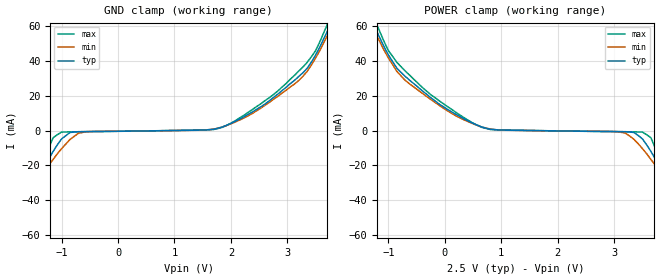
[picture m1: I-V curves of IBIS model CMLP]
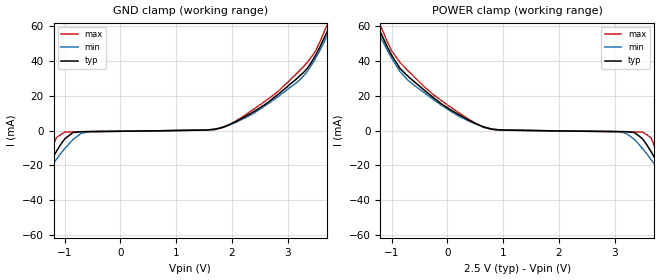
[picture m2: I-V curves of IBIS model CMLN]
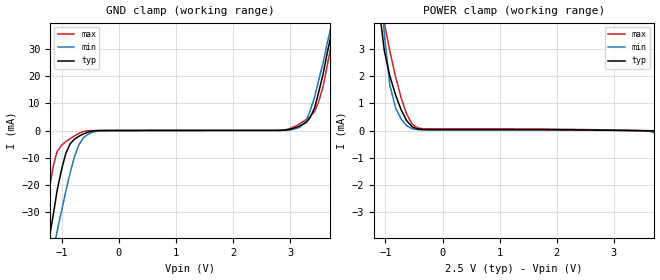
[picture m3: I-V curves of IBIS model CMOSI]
|   Texas Instruments Incorporated
|   IBIS Model of DS30EA101
[IBIS Ver]   4.2
[File name]   ds30ea101.ibs
[File Rev]   1.0
[Date]   2/15/2012
[Source]   Generated by Texas Instruments Incorporated
[Notes]   Created By Pegah Alavi
[Disclaimer]
  This model is designed as an aid for customers of Texas Instruments.
  TI and its licensors and suppliers make no warranties, either expressed
  or implied, with respect to this model, including the warranties of
  merchantability or fitness for a particular purpose.  The model is
  provided solely on an "as is" basis.  The entire risk as to its quality
  and performance is with the customer.
[Copyright] (C) Copyright 2012 Texas Instruments Incorporated.
   All rights reserved.
[Component]   DS30EA101
[Manufacturer]  Texas Instruments
[Package]
|   typ   min   max
R_pkg   0   0   0
L_pkg   0   0   0
C_pkg   0   0   0
[Pin]   signal_name   model_name   R_pin   L_pin   C_pin
1   VEE   GND
2   IN   CMLP
3   INb   CMLN
4   VEE   GND
5   DNC   NC
6   DNC   NC
7   VEE   GND
8   VEE   GND
9   VEE   GND
10   OUTb   LVDSN
11   OUT   LVDSP
12   VEE   GND
13   VCC   POWER
14   ENb   CMOSI
15   LOS   NC
16   VCC   POWER
17   DAP   GND
[Package Model]  llp16_ds30ea101
[Diff pin]  inv_pin  vdiff  tdelay_typ  tdelay_min  tdelay_max
2   3   2.5   0.0s   0.0s   0.0s
11   10   0.0   0.0s   0.0s   0.0s
[Define Package Model]  llp16_ds30ea101
[Manufacturer]  Unknown
[OEM]  Unknown
[Description]  Package Model at 1.5GHz
[Number Of Pins]  17
[Pin Numbers]
17   | 17 = DAP
1   | 1 = L1
2   | 2 = L2
3   | 3 = L3
4   | 4 = L4
5   | 5 = L5
6   | 6 = L6
7   | 7 = L7
8   | 8 = L8
9   | 9 = L9
10   | 10 = L10
11   | 11 = L11
12   | 12 = L12
13   | 13 = L13
14   | 14 = L14
15   | 15 = L15
16   | 16 = L16
[Model Data]
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[End Model Data]
[End Package Model]
| Models and submodels in the file (5): CMLP (Input), CMLN (Input), CMOSI (Input), LVDSP (Output), LVDSN (Output)
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|   Model CMLP
[Model]  CMLP
Model_type Input
Polarity   Non-Inverting
Vinl =   0
Vinh =   2
C_comp   914fF   914fF   914fF
[Temperature Range]   25.000   85.000   -40.000
[Voltage Range]   2.500V   2.3750V   2.6250V
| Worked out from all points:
|   GND clamp passes 1 mA (typ) near -0.81 V on its own axis
[GND_clamp]
|Voltage   I(typ)   I(min)   I(max)
-2.5V     -115mA     -97mA      -177mA
-1.98V    -69mA      -62mA      -99.9mA
-1.83V    -56.8mA    -52.4mA    -80mA
-1.68V    -45.5mA    -43.2mA    -60.8mA
-1.23V    -16.4mA    -19.9mA    -10.3mA
-1V       -4.8mA     -10.4mA    -899uA
-550mV    -604uA     -609uA     -663uA
1.85V     2.04mA     2.06mA     1.85mA
3.2V      30.9mA     28.6mA     34mA
3.73V     58.3mA     55.6mA     62.4mA
3.8V      63.7mA     60.5mA     68.4mA
5V        183mA      164mA      211mA
[POWER_clamp]
|Voltage   I(typ)   I(min)   I(max)
-2.5V     183mA      164mA      211mA
-1.3V     63.7mA     60.5mA     68.4mA
-1.23V    58.3mA     55.6mA     62.4mA
-700mV    30.9mA     28.6mA     34mA
650mV     2.04mA     2.06mA     1.85mA
3.05V     -604uA     -609uA     -663uA
3.5V      -4.8mA     -10.4mA    -899uA
3.73V     -16.4mA    -19.9mA    -10.3mA
4.18V     -45.5mA    -43.2mA    -60.8mA
4.33V     -56.8mA    -52.4mA    -80mA
4.48V     -69mA      -62mA      -99.9mA
5V        -115mA     -97mA      -177mA
|   Model CMLN
[Model]  CMLN
Model_type Input
Polarity   Inverting
Vinl =   0
Vinh =   2
C_comp   914fF   914fF   914fF
[Temperature Range]   25.000   85.000   -40.000
[Voltage Range]   2.500V   2.3750V   2.6250V
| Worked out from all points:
|   GND clamp passes 1 mA (typ) near -0.81 V on its own axis
[GND_clamp]
|Voltage   I(typ)   I(min)   I(max)
-2.5V     -115mA     -97mA      -177mA
-1.98V    -69mA      -62mA      -99.9mA
-1.83V    -56.8mA    -52.4mA    -80mA
-1.68V    -45.5mA    -43.2mA    -60.8mA
-1.23V    -16.4mA    -19.9mA    -10.3mA
-1V       -4.8mA     -10.4mA    -899uA
-550mV    -604uA     -609uA     -663uA
1.85V     2.04mA     2.06mA     1.85mA
3.2V      30.9mA     28.6mA     34mA
3.73V     58.3mA     55.6mA     62.4mA
3.8V      63.7mA     60.5mA     68.4mA
5V        183mA      164mA      211mA
[POWER_clamp]
|Voltage   I(typ)   I(min)   I(max)
-2.5V     183mA      164mA      211mA
-1.3V     63.7mA     60.5mA     68.4mA
-1.23V    58.3mA     55.6mA     62.4mA
-700mV    30.9mA     28.6mA     34mA
650mV     2.04mA     2.06mA     1.85mA
3.05V     -604uA     -609uA     -663uA
3.5V      -4.8mA     -10.4mA    -899uA
3.73V     -16.4mA    -19.9mA    -10.3mA
4.18V     -45.5mA    -43.2mA    -60.8mA
4.33V     -56.8mA    -52.4mA    -80mA
4.48V     -69mA      -62mA      -99.9mA
5V        -115mA     -97mA      -177mA
|   Model CMOSI
[Model]  CMOSI
Model_type Input
Vinl =   0
Vinh =   2
C_comp   914fF   914fF   914fF
[Temperature Range]   25.000   85.000   -40.000
[Voltage Range]   2.500V   2.3750V   2.6250V
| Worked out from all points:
|   GND clamp passes 1 mA (typ) near -0.59 V on its own axis
|   POWER clamp passes 1 mA (typ) near -0.77 V on its own axis
[GND_clamp]
|Voltage   I(typ)   I(min)   I(max)
-2.5V     -233mA     -200mA     -336mA
-1.38V    -61.8mA    -69.1mA    -53.1mA
-1.3V     -51.3mA    -60.9mA    -37.1mA
-1.23V    -41mA      -52.7mA    -23.3mA
-1.08V    -22mA      -36.9mA    -7.71mA
-925mV    -8.19mA    -22mA      -4.04mA
-700mV    -2.12mA    -5.3mA     -1.04mA
2.98V     356uA      174uA      595uA
3.43V     8.28mA     12.3mA     6.89mA
3.73V     36.1mA     39.1mA     32.2mA
3.8V      44.3mA     46.4mA     41.3mA
5V        184mA      172mA      201mA
[POWER_clamp]
|Voltage   I(typ)   I(min)   I(max)
-3.3V     184mA      172mA      201mA
-1.12V    4.67mA     7.12mA     5.12mA
-1.02V    2.93mA     3.53mA     3.95mA
-924mV    2.01mA     1.67mA     2.93mA
-825mV    1.32mA     850uA      2mA
-528mV    133uA      64.3uA     227uA
3.73V     -19.3uA    -94.8uA    -12.1uA
4.03V     -653uA     -1.48mA    -101uA
4.22V     -2.12mA    -5.3mA     -1.04mA
4.42V     -4.83mA    -15.3mA    -2.95mA
4.52V     -8.19mA    -22mA      -4.04mA
6.6V      -233mA     -200mA     -336mA
